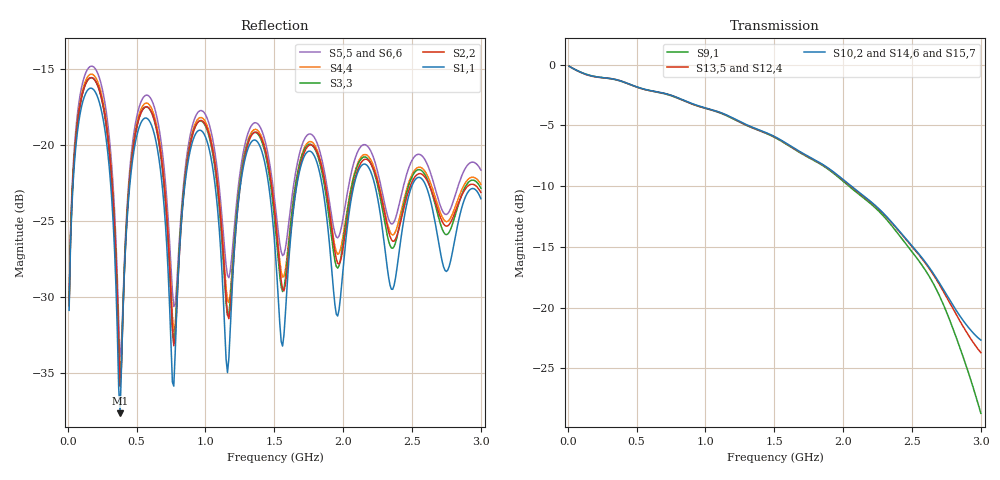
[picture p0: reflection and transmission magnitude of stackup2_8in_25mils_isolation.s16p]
! Touchstone file from project
# GHZ S RI R 50.000000
! Modal data exported
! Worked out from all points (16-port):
!   300 points, 10 MHz to 3 GHz, reference 50 ohm
!   strongest paths, dB at 10 MHz, 760 MHz, 1.51 GHz, 2.26 GHz, 3 GHz:
!     S10,2: -0.1, -2.5, -6.0, -11.9, -22.7
!     S13,5: -0.1, -2.6, -6.0, -11.9, -23.7
!     S14,6: -0.1, -2.6, -6.0, -11.9, -23.1
!     S12,4: -0.1, -2.6, -6.0, -12.0, -23.3
!     S15,7: -0.1, -2.6, -6.0, -12.0, -22.7
!     S9,1: -0.1, -2.6, -6.0, -12.1, -28.7
!   lowest |S11| = -37.7 dB at 380 MHz (marker M1), VSWR 1.03, Z = 51.3 - j0.0714 ohm
!   |S11| at or under -10 dB: start of sweep to end of sweep
